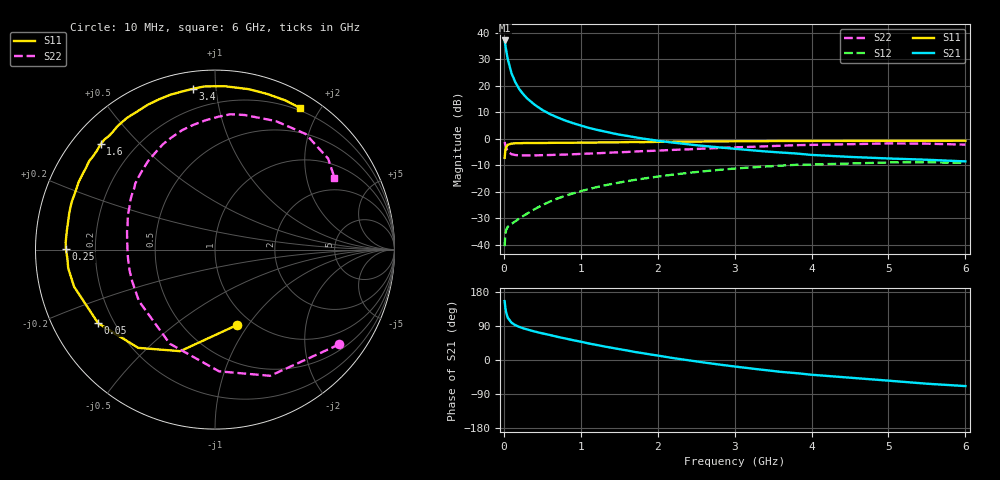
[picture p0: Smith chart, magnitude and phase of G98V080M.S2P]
! SIEMENS Small Signal Semiconductors
! BFG235
! Si NPN RF Bipolar Junction Transistor in SOT223
! VCE = 8 V  IC = 80 mA
! Common Emitter S-Parameters:  July  1994
# GHz  S  MA  R  50
!  f  S11  S21  S12  S22
! GHz  MAG  ANG  MAG  ANG  MAG  ANG  MAG  ANG
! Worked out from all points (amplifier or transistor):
!   40 points, 10 MHz to 6 GHz, reference 50 ohm
!   highest |S21| = 37.0 dB at 10 MHz (marker M1)
!   |S21| within 3 dB of that: start of sweep to 26.59 MHz
!   unconditionally stable (mu >= 1): 491.9 MHz to 1.47 GHz
!   at 200 MHz: K = 0.74, MSG = 24.4 dB, |S12| = -30.0 dB
!   at 1.5 GHz: K = 1.00, MSG = 9.0 dB, |S12| = -16.5 dB
!   at 6 GHz: K = 0.89, MSG = 0.3 dB, |S12| = -9.1 dB
!   S11 on the Smith chart (normalised r, x): 10 MHz: 0.85, -0.89; 50 MHz: 0.14, -0.28; 250 MHz: 0.09, +0.00; 1.6 GHz: 0.08, +0.39; 3.4 GHz: 0.09, +0.87; 6 GHz: 0.17, +1.76
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0.01  0.4378 -73.8  71.17 155.4  0.0095 67.4  0.8711 -37.3
0.02  0.598 -108.9  58.03 137.4  0.0158 52.2  0.7673 -66.4
0.03  0.6948 -128.0  46.83 125.4  0.0191 44.3  0.6786 -88.1
0.05  0.7695 -147.8  32 111.9  0.022 34.7  0.5816 -115.7
0.1  0.8121 -165.3  17.14 98.4  0.0251 34.2  0.5118 -145.9
0.15  0.8243 -172.8  11.55 91.8  0.0279 38.5  0.4942 -158.9
0.2  0.8241 -176.7  8.659 87.5  0.0316 42.5  0.49 -166.1
0.25  0.8308 179.8  6.976 83.8  0.035 46.0  0.4874 -171.0
0.3  0.8331 177.2  5.826 80.8  0.0388 49.0  0.4871 -175.0
0.4  0.8319 172.5  4.384 75.2  0.0473 52.9  0.4876 179.6
0.5  0.8336 168.6  3.498 70.3  0.0565 54.7  0.4909 175.3
0.6  0.8378 165.5  2.918 65.9  0.0658 55.5  0.4953 171.4
0.7  0.8413 161.8  2.516 61.0  0.0753 55.6  0.5007 168.1
0.9  0.8432 156.2  1.969 52.3  0.0938 53.8  0.5112 162.1
1.1  0.8494 149.9  1.612 43.8  0.1127 51.3  0.5262 156.3
1.6  0.8666 137.3  1.136 25.2  0.159 42.3  0.5646 142.9
2.2  0.8827 123.8  0.847 5.1  0.2114 29.7  0.6184 127.0
3.2  0.8994 102.1  0.612 -22.0  0.2879 6.6  0.7044 100.2
3.4  0.9042 97.9  0.578 -26.7  0.3004 1.7  0.7217 94.4
4.5  0.9135 78.0  0.456 -46.7  0.343 -23.9  0.792 64.7
5.5  0.9188 64.9  0.403 -62.6  0.3619 -46.2  0.809 38.8
6  0.9209 58.9  0.375 -68.8  0.3512 -54.6  0.7768 31.1
